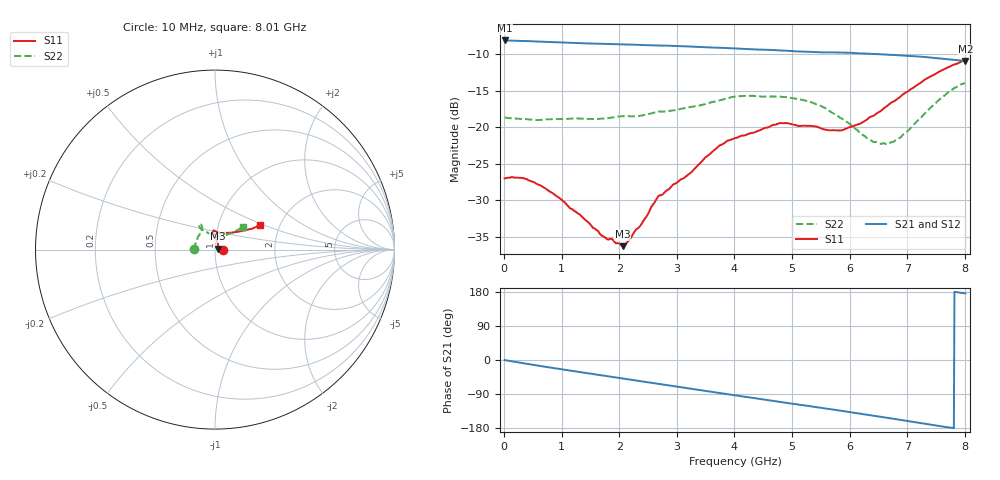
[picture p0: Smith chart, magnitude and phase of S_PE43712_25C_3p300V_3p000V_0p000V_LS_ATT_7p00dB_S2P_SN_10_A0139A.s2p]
! DEVICE ID: PE43712
! File Path: z:\PE43713\PE43713_CHAR_NOM_04292014\AMB\3p300\LS_ATT_7p00dB\PE43713_AMB_3p300V_3p000V_0p000V_LS_ATT_7p00dB_S2P_SN_10_A0139A.s2p
! Serial: 10
! Lot: A0139A
! Temp: 25C
! VDD: 3.300
! VSS: 0.000
! Control_Hi: 3.000
! Control_Lo: 0.000
! Attenuation Step: 7.00dB
! Port 1: RF1
! Port 2: RF2
! ThroughPath:1-2
! IDD: 0.0001474126
! ISS: -8.97e-008
#  Hz  S  RI  R  50
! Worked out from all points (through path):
!   801 points, 10 MHz to 8.01 GHz, reference 50 ohm
!   highest |S21| = -8.14 dB at 10 MHz (marker M1); lowest = -10.9 dB at 8.01 GHz (marker M2)
!   group delay of S21, straight-line fit = 63.2 ps
!   lowest |S11| = -36.3 dB at 2.06 GHz (marker M3), VSWR 1.03, Z = 51.4 + j0.58 ohm
!   |S11| at or under -10 dB: start of sweep to end of sweep
!   |S22| runs from -22.3 to -14.0 dB; largest |S21 - S12| = 0.0013
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1e7  0.0446 -5.77e-05  0.3919 -0.00215  0.3918 -0.00216  -0.1166 0.000721
3e8  0.0444 -0.00731  0.3855 -0.0528  0.3854 -0.0528  -0.1134 0.0101
5.4e8  0.0401 -0.011  0.3748 -0.0915  0.3749 -0.0916  -0.1107 0.017
9.6e8  0.0305 -0.0121  0.3479 -0.1529  0.348 -0.1529  -0.1093 0.0308
1.35e9  0.0227 -0.00921  0.316 -0.2022  0.316 -0.2023  -0.1059 0.0431
1.71e9  0.0179 -0.00266  0.2813 -0.2427  0.2813 -0.2426  -0.0993 0.0565
2.06e9  0.0143 0.00564  0.2429 -0.277  0.243 -0.2768  -0.0957 0.0706
2.15e9  0.0147 0.00766  0.2323 -0.2849  0.2323 -0.2847  -0.0936 0.0735
2.38e9  0.0148 0.0157  0.2037 -0.3031  0.2037 -0.303  -0.0859 0.0836
2.68e9  0.0169 0.0292  0.1652 -0.3216  0.1652 -0.3217  -0.0773 0.1018
3.23e9  0.00964 0.0473  0.0892 -0.3446  0.0892 -0.3447  -0.0729 0.1162
3.72e9  0.00499 0.0735  0.0211 -0.3489  0.0209 -0.3488  -0.074 0.1328
4.01e9  -0.000445 0.0842  -0.019 -0.3453  -0.019 -0.3452  -0.0812 0.1402
4.79e9  -0.00858 0.1064  -0.1176 -0.3136  -0.1177 -0.3139  -0.0883 0.1358
5.35e9  0.00213 0.1016  -0.1772 -0.275  -0.1771 -0.2748  -0.0845 0.1209
5.63e9  0.0138 0.0943  -0.2035 -0.2532  -0.2034 -0.2533  -0.0701 0.1099
5.88e9  0.0273 0.0916  -0.2276 -0.2304  -0.2271 -0.2304  -0.0531 0.1008
6.4e9  0.0731 0.0939  -0.2647 -0.1744  -0.2643 -0.1742  -0.00847 0.0794
6.68e9  0.1054 0.0963  -0.2794 -0.1407  -0.279 -0.1407  0.0205 0.0743
6.99e9  0.1405 0.1023  -0.2911 -0.1021  -0.2907 -0.1021  0.0505 0.0777
7.7e9  0.2237 0.1242  -0.2917 -0.0131  -0.2914 -0.0134  0.1305 0.1121
8.01e9  0.2529 0.1377  -0.2829 0.0202  -0.2824 0.0198  0.1542 0.128
